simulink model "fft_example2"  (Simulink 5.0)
settings: Solver=ode45  StartTime=0.0  StopTime=10000.0  RelTol=1e-3
undefined symbols (not defined in the file or in its folder): get, hamming, N, tmp5
libraries: xbsIndex_r3 x50, xrbsControl_r3 x4, ADlibrary x3, dspsigattribs x2, dspsnks4 x2, simulink x1

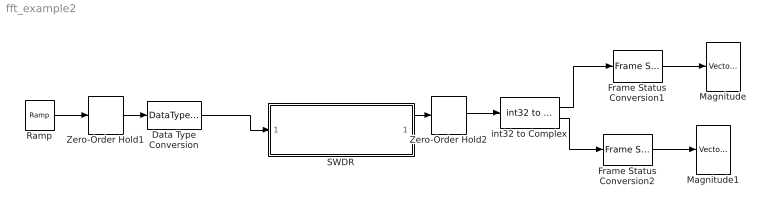
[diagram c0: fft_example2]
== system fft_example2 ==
  Data Type Conversion : DataTypeConversion  DataType=uint32
  Frame Status Conversion1 : dspsigattribs/Frame Status Conversion  growRefPort=off  outframe=Frame-based
  Frame Status Conversion2 : dspsigattribs/Frame Status Conversion  growRefPort=off  outframe=Frame-based
  Magnitude : dspsnks4/Vector Scope  ScopeProperties=on  Domain=User-defined  HorizSpan=1  DisplayProperties=off  AxisGrid=on  Memory=off  FrameNumber=on  AxisLegend=off  AxisZoom=off  OpenScopeAtSimStart=on  OpenScopeImmediately=off  FigPos=get(0,'defaultfigureposition')  AxisProperties=off  XUnits=Hertz  XRange=[0...Fs/2]  InheritXIncr=on  XIncr=1  XLabel=Frequency  YUnits=dB  YLabel=Magnitude  LineProperties=off
  Magnitude1 : dspsnks4/Vector Scope  ScopeProperties=on  Domain=User-defined  HorizSpan=1  DisplayProperties=off  AxisGrid=on  Memory=off  FrameNumber=on  AxisLegend=off  AxisZoom=off  OpenScopeAtSimStart=on  OpenScopeImmediately=off  FigPos=get(0,'defaultfigureposition')  AxisProperties=off  XUnits=Hertz  XRange=[0...Fs/2]  InheritXIncr=on  XIncr=1  XLabel=Frequency  YUnits=dB  YLabel=Magnitude  LineProperties=off
  Ramp : simulink/Sources/Ramp  slope=.02  start=0  X0=8
  SWDR : Subsystem
  Zero-Order Hold1 : ZeroOrderHold
  Zero-Order Hold2 : ZeroOrderHold  SampleTime=370
  int32 to Complex : ADlibrary/Miscellaneous/int32 to Complex
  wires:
  Frame Status Conversion1/1 -> Magnitude/1
  Ramp/1 -> Zero-Order Hold1/1
  Zero-Order Hold1/1 -> Data Type Conversion/1
  Data Type Conversion/1 -> SWDR/1(Vector Input)
  SWDR/1(Vector Output) -> Zero-Order Hold2/1
  Zero-Order Hold2/1 -> int32 to Complex/1
  Frame Status Conversion2/1 -> Magnitude1/1
  int32 to Complex/1 -> Frame Status Conversion1/1
  int32 to Complex/2 -> Frame Status Conversion2/1

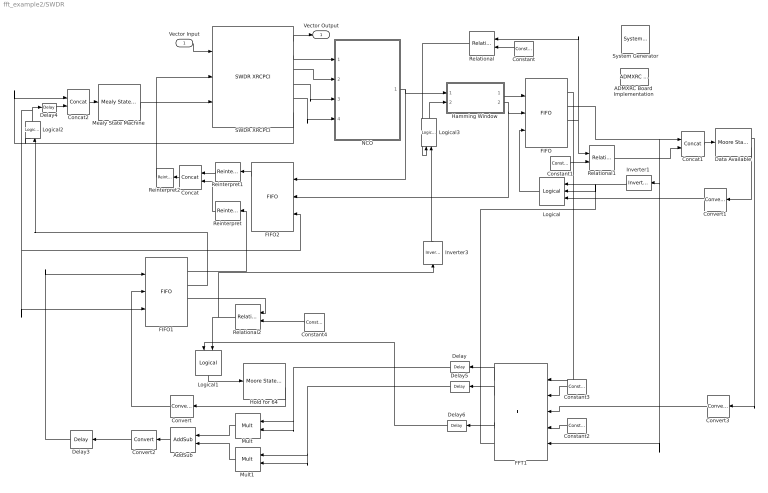
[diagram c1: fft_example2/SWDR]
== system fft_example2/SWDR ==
  Vector Input : Inport
  " System Generator" : xbsIndex_r3/ System Generator  Tag=genX  xilinxfamily=Virtex2  part=xc2v6000  speed=-4  package=ff1152  synthesis_tool=XST  directory=e:/tmp5  testbench=off  simulink_period=1  sysclk_period=15  incr_netlist=off  trim_vbits=According to Block Masks  dbl_ovrd=According to Block Masks  core_generation=According to Block Masks  run_coregen=off  deprecated_control=off  eval_field=0
  ADMXRC Board  Implementation : ADlibrary/Miscellaneous/ADMXRC Board  Implementation  board=XRCII  run_synth=on  make_clean=off  lvds_io_std=3.3v  clock_source=MCLK
  AddSub : xbsIndex_r3/AddSub  Orientation=left  mode=Addition  precision=Full  arith_type=Unsigned  n_bits=8  bin_pt=2  quantization=Truncate  overflow=Wrap  latency=0  explicit_period=off  period=1  en=off  dbl_ovrd=off  use_core=on  pipeline=off  use_rpm=off  gen_core=on
  Concat : xbsIndex_r3/Concat  Orientation=left  num_inputs=2  explicit_period=off  period=1  dbl_ovrd=off
  Concat1 : xbsIndex_r3/Concat  num_inputs=2  explicit_period=off  period=1  dbl_ovrd=off
  Concat2 : xbsIndex_r3/Concat  num_inputs=2  explicit_period=off  period=1  dbl_ovrd=off
  Constant : xbsIndex_r3/Constant  Orientation=left  const=.75  arith_type=Unsigned  n_bits=3  bin_pt=3  explicit_period=off  period=1  dbl_ovrd=off
  Constant1 : xbsIndex_r3/Constant  const=.25  arith_type=Unsigned  n_bits=3  bin_pt=3  explicit_period=off  period=1  dbl_ovrd=off
  Constant2 : xbsIndex_r3/Constant  Orientation=left  const=0  arith_type=Boolean  n_bits=1  bin_pt=0  explicit_period=on  period=1  dbl_ovrd=off
  Constant3 : xbsIndex_r3/Constant  Orientation=left  const=0  arith_type="Signed  (2's comp)"  n_bits=16  bin_pt=0  explicit_period=on  period=1  dbl_ovrd=off
  Constant4 : xbsIndex_r3/Constant  Orientation=left  const=.7  arith_type=Unsigned  n_bits=5  bin_pt=5  explicit_period=off  period=1  dbl_ovrd=off
  Convert : xbsIndex_r3/Convert  Orientation=left  arith_type=Boolean  n_bits=8  bin_pt=6  quantization=Truncate  overflow=Wrap  latency=0  explicit_period=off  period=1  dbl_ovrd=off  inserted_by_tool=off
  Convert1 : xbsIndex_r3/Convert  Orientation=left  arith_type=Boolean  n_bits=8  bin_pt=6  quantization=Truncate  overflow=Wrap  latency=0  explicit_period=off  period=1  dbl_ovrd=off  inserted_by_tool=off
  Convert2 : xbsIndex_r3/Convert  Orientation=left  arith_type="Signed  (2's comp)"  n_bits=16  bin_pt=0  quantization=Truncate  overflow=Wrap  latency=0  explicit_period=off  period=1  dbl_ovrd=off  inserted_by_tool=off
  Convert3 : xbsIndex_r3/Convert  Orientation=left  arith_type=Boolean  n_bits=8  bin_pt=6  quantization=Truncate  overflow=Wrap  latency=0  explicit_period=off  period=1  dbl_ovrd=off  inserted_by_tool=off
  Data Available : xrbsControl_r3/Moore State Machine  next_state_matrix=[0 1 0 1;1 1 0 0]  output_matrix=[0;1]  n_bits=1  period=1
  Delay : xbsIndex_r3/Delay  Orientation=left  latency=1  reg_retiming=off  explicit_period=on  period=1  en=off  accept_only_valid=off  init_zero=on  dbl_ovrd=off
  Delay3 : xbsIndex_r3/Delay  Orientation=left  latency=1  reg_retiming=off  explicit_period=on  period=1  en=off  accept_only_valid=off  init_zero=on  dbl_ovrd=off
  Delay4 : xbsIndex_r3/Delay  latency=1  reg_retiming=off  explicit_period=on  period=1  en=off  accept_only_valid=off  init_zero=on  dbl_ovrd=off
  Delay5 : xbsIndex_r3/Delay  Orientation=left  latency=1  reg_retiming=off  explicit_period=on  period=1  en=off  accept_only_valid=off  init_zero=on  dbl_ovrd=off
  Delay6 : xbsIndex_r3/Delay  Orientation=left  latency=2  reg_retiming=off  explicit_period=on  period=1  en=off  accept_only_valid=off  init_zero=on  dbl_ovrd=off
  FFT1 : xbsIndex_r3/FFT  Orientation=left  n=64  mem=Single  scale_mode=1/N  oflw_inv=off  explicit_period=on  period=1  rst=on  dbl_ovrd=off  gen_core=on
  FIFO : xbsIndex_r3/FIFO  depth=256  percent_nbits=3  mem_type=Block RAM  store_only_valid=on  init_zero=on  explicit_period=on  period=1  rst=off  en=off  dbl_ovrd=off  gen_core=on
  FIFO1 : xbsIndex_r3/FIFO  depth=512  percent_nbits=5  mem_type=Block RAM  store_only_valid=off  init_zero=on  explicit_period=on  period=1  rst=off  en=off  dbl_ovrd=off  gen_core=on
  FIFO2 : xbsIndex_r3/FIFO  Orientation=left  depth=1K  percent_nbits=3  mem_type=Block RAM  store_only_valid=on  init_zero=on  explicit_period=on  period=1  rst=off  en=off  dbl_ovrd=off  gen_core=on
  Hamming Window : Subsystem
  Hold for 64 : xrbsControl_r3/Moore State Machine  next_state_matrix=[0 1;[(2:64)' (2:64)']; 0 0]  output_matrix=[0;ones(64,1)]  n_bits=1  period=1
  Inverter1 : xbsIndex_r3/Inverter  Orientation=left  latency=0  explicit_period=off  period=1  en=off  dbl_ovrd=off
  Inverter3 : xbsIndex_r3/Inverter  Orientation=up  latency=0  explicit_period=off  period=1  en=off  dbl_ovrd=off
  Logical : xbsIndex_r3/Logical  Orientation=left  logical_function=AND  inputs=3  precision=Full  arith_type=Unsigned  n_bits=8  bin_pt=2  align_bp=on  latency=0  explicit_period=off  period=1  en=off  dbl_ovrd=off
  Logical1 : xbsIndex_r3/Logical  Orientation=down  logical_function=AND  inputs=2  precision=Full  arith_type=Unsigned  n_bits=8  bin_pt=2  align_bp=on  latency=0  explicit_period=off  period=1  en=off  dbl_ovrd=off
  Logical2 : xbsIndex_r3/Logical  Orientation=up  logical_function=NOR  inputs=2  precision=Full  arith_type=Unsigned  n_bits=8  bin_pt=2  align_bp=on  latency=0  explicit_period=off  period=1  en=off  dbl_ovrd=off
  Logical3 : xbsIndex_r3/Logical  Orientation=up  logical_function=OR  inputs=2  precision=Full  arith_type=Unsigned  n_bits=8  bin_pt=2  align_bp=on  latency=0  explicit_period=off  period=1  en=off  dbl_ovrd=off
  Mealy State Machine : xrbsControl_r3/Mealy State Machine  next_state_matrix=[0 0 1 1; 0 0 1 1]  output_matrix=[0 1 0 0; 1 1 0 0]  n_bits=1  period=1
  Mult : xbsIndex_r3/Mult  Orientation=left  precision=Full  arith_type="Signed  (2's comp)"  n_bits=16  bin_pt=0  quantization=Truncate  overflow=Wrap  mult_type=Parallel  use_embedded=off  pipeline=off  latency=1  explicit_period=off  period=1  en=off  dbl_ovrd=off  oversample=2  use_rpm=off  placement_style=Rectangular Shape  gen_core=on
  Mult1 : xbsIndex_r3/Mult  Orientation=left  precision=Full  arith_type="Signed  (2's comp)"  n_bits=16  bin_pt=0  quantization=Truncate  overflow=Wrap  mult_type=Parallel  use_embedded=off  pipeline=off  latency=1  explicit_period=off  period=1  en=off  dbl_ovrd=off  oversample=2  use_rpm=off  placement_style=Rectangular Shape  gen_core=on
  NCO : Subsystem
  Reinterpret : xbsIndex_r3/Reinterpret  Orientation=left  force_arith_type=on  arith_type=Unsigned  force_bin_pt=on  bin_pt=0  force_valid=off
  Reinterpret1 : xbsIndex_r3/Reinterpret  Orientation=left  force_arith_type=on  arith_type=Unsigned  force_bin_pt=on  bin_pt=0  force_valid=off
  Reinterpret2 : xbsIndex_r3/Reinterpret  Orientation=left  force_arith_type=on  arith_type="Signed  (2's comp)"  force_bin_pt=on  bin_pt=0  force_valid=off
  Relational : xbsIndex_r3/Relational  Orientation=left  mode=a>=b  latency=0  explicit_period=off  period=1  en=off  dbl_ovrd=off
  Relational1 : xbsIndex_r3/Relational  mode=a>=b  latency=0  explicit_period=off  period=1  en=off  dbl_ovrd=off
  Relational2 : xbsIndex_r3/Relational  Orientation=left  mode=a<b  latency=0  explicit_period=off  period=1  en=off  dbl_ovrd=off
  SWDR XRCPCI : ADlibrary/PCI/SWDR XRCPCI  AncestorBlock=ADlibrary/PCI/ADMA XRCPCI  no_inputs=1  no_outputs=64  circuit_lag=192  fifo_length=256  debug=0
  Vector Output : Outport
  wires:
  SWDR XRCPCI/1 -> Vector Output/1
  Vector Input/1 -> SWDR XRCPCI/1
  SWDR XRCPCI/2 -> NCO/1(data)
  SWDR XRCPCI/3 -> NCO/2(addr)
  SWDR XRCPCI/5 -> NCO/4(reset)
  NCO/1(sine) -> Hamming Window/1(data), FIFO2/1
  Hamming Window/1(wdata) -> FIFO/1
  Constant/1 -> Relational/2
  Constant1/1 -> Relational1/2
  FIFO/2 -> Concat1/1, Inverter1/1, FFT1/5
  Inverter1/1 -> Logical/1
  Mult/1 -> AddSub/1
  Mult1/1 -> AddSub/2
  AddSub/1 -> Convert2/1
  Delay3/1 -> FIFO1/1
  Logical1/1 -> Hold for 64/1
  Constant4/1 -> Relational2/2
  Delay6/1 -> Logical1/1
  FIFO1/1 -> Reinterpret/1
  Reinterpret1/1 -> Concat/1
  Reinterpret/1 -> Concat/2
  Concat/1 -> Reinterpret2/1
  Relational1/1 -> Concat1/2
  Concat1/1 -> Data Available/1
  Data Available/2 -> Convert1/1
  Logical3/1 -> Hamming Window/2(wait)
  Inverter3/1 -> Logical3/2
  Relational/1 -> Logical3/1
  SWDR XRCPCI/4 -> NCO/3(write)
  Hamming Window/2(write) -> FIFO/2, FIFO2/2
  Logical/1 -> FIFO/3
  Reinterpret2/1 -> SWDR XRCPCI/2
  FIFO2/1 -> Reinterpret1/1
  Concat2/1 -> Mealy State Machine/1
  Mealy State Machine/2 -> SWDR XRCPCI/3
  SWDR XRCPCI/6 -> Concat2/1, Logical2/1
  Delay4/1 -> Concat2/2
  Logical2/1 -> Delay4/1, FIFO1/3, FIFO2/3
  Convert2/1 -> Delay3/1
  FIFO1/3 -> Relational2/1
  Relational2/1 -> Logical1/2, Inverter3/1
  Hold for 64/2 -> Convert/1
  FIFO/3 -> Relational/1, Relational1/1
  FFT1/1 -> Delay/1
  FFT1/2 -> Delay5/1
  FFT1/4 -> Delay6/1
  FFT1/5 -> Logical/2
  Constant3/1 -> FFT1/2
  FIFO/1 -> FFT1/1
  Constant2/1 -> FFT1/4
  Data Available/1 -> Convert3/1
  FIFO1/2 -> Logical2/2
  Delay/1 -> Mult/1, Mult/2
  Delay5/1 -> Mult1/1, Mult1/2
  Convert/1 -> FIFO1/2
  Convert1/1 -> Logical/3
  Convert3/1 -> FFT1/3

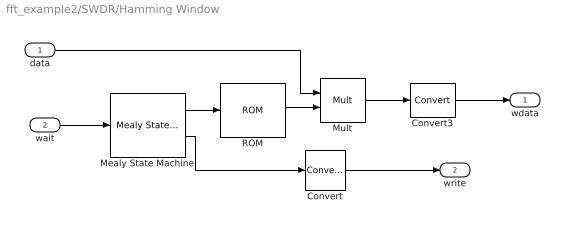
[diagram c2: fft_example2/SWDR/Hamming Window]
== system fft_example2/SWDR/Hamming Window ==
  data : Inport
  wait : Inport  Port=2
  Convert : xbsIndex_r3/Convert  arith_type=Boolean  n_bits=8  bin_pt=6  quantization=Truncate  overflow=Wrap  latency=0  explicit_period=off  period=1  dbl_ovrd=off  inserted_by_tool=off
  Convert3 : xbsIndex_r3/Convert  arith_type="Signed  (2's comp)"  n_bits=16  bin_pt=0  quantization=Truncate  overflow=Wrap  latency=0  explicit_period=on  period=1  dbl_ovrd=off  inserted_by_tool=off
  Mealy State Machine : xrbsControl_r3/Mealy State Machine  next_state_matrix=[1 0;[(2:63)' (2:63)'];0 0]  output_matrix=[1 0;ones(63,2)]  n_bits=1  period=1
  Mult : xbsIndex_r3/Mult  precision=Full  arith_type="Signed  (2's comp)"  n_bits=8  bin_pt=2  quantization=Truncate  overflow=Wrap  mult_type=Parallel  use_embedded=off  pipeline=off  latency=0  explicit_period=on  period=1  en=off  dbl_ovrd=off  oversample=2  use_rpm=off  placement_style=Rectangular Shape  gen_core=on
  ROM : xbsIndex_r3/ROM  depth=64  initVector=hamming(64)  arith_type="Signed  (2's comp)"  n_bits=16  bin_pt=16  latency=1  distributed_mem=off  init_zero=on  explicit_period=on  period=1  rst=off  init_reg=0  en=off  dbl_ovrd=off  use_rpm=off  gen_core=on
  wdata : Outport
  write : Outport  Port=2
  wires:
  wait/1 -> Mealy State Machine/1
  Mealy State Machine/1 -> ROM/1
  ROM/1 -> Mult/2
  data/1 -> Mult/1
  Mult/1 -> Convert3/1
  Mealy State Machine/2 -> Convert/1
  Convert3/1 -> wdata/1
  Convert/1 -> write/1

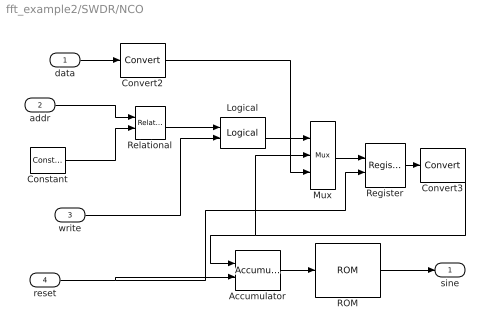
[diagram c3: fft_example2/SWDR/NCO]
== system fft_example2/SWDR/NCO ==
  data : Inport
  addr : Inport  Port=2
  write : Inport  Port=3
  reset : Inport  Port=4
  Accumulator : xbsIndex_r3/Accumulator  n_bits=10  overflow=Wrap  operation=Add  scale=1  explicit_period=off  period=1  rst=on  hasbypass=on  en=off  dbl_ovrd=off  gen_core=on  use_rpm=off
  Constant : xbsIndex_r3/Constant  const=0  arith_type=Unsigned  n_bits=22  bin_pt=0  explicit_period=on  period=1  dbl_ovrd=off
  Convert2 : xbsIndex_r3/Convert  arith_type=Unsigned  n_bits=10  bin_pt=0  quantization=Truncate  overflow=Wrap  latency=0  explicit_period=on  period=1  dbl_ovrd=off  inserted_by_tool=off
  Convert3 : xbsIndex_r3/Convert  arith_type=Unsigned  n_bits=10  bin_pt=0  quantization=Truncate  overflow=Wrap  latency=0  explicit_period=on  period=1  dbl_ovrd=off  inserted_by_tool=off
  Logical : xbsIndex_r3/Logical  logical_function=AND  inputs=2  precision=Full  arith_type=Unsigned  n_bits=8  bin_pt=2  align_bp=on  latency=0  explicit_period=on  period=1  en=off  dbl_ovrd=off
  Mux : xbsIndex_r3/Mux  inputs=2  precision=Full  arith_type="Signed  (2's comp)"  n_bits=8  bin_pt=2  quantization=Truncate  overflow=Wrap  latency=0  mux_type=off  explicit_period=on  period=1  en=off  dbl_ovrd=off  use_rpm=off  gen_core=on
  ROM : xbsIndex_r3/ROM  depth=1024  initVector=256*sin(2*pi*(0:1023)/1024)  arith_type="Signed  (2's comp)"  n_bits=16  bin_pt=0  latency=1  distributed_mem=off  init_zero=on  explicit_period=on  period=1  rst=off  init_reg=0  en=off  dbl_ovrd=off  use_rpm=off  gen_core=on
  Register : xbsIndex_r3/Register  init=0  reg_only_valid=on  explicit_period=on  period=1  rst=on  en=off  out_en=off  dbl_ovrd=off
  Relational : xbsIndex_r3/Relational  mode=a=b  latency=0  explicit_period=on  period=1  en=off  dbl_ovrd=off
  sine : Outport
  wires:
  Accumulator/1 -> ROM/1
  data/1 -> Convert2/1
  Register/1 -> Convert3/1
  Mux/1 -> Register/1
  Convert3/1 -> Accumulator/1, Mux/2
  Convert2/1 -> Mux/3
  Logical/1 -> Mux/1
  write/1 -> Logical/2
  Constant/1 -> Relational/2
  addr/1 -> Relational/1
  ROM/1 -> sine/1
  reset/1 -> Accumulator/2, Register/2
  Relational/1 -> Logical/1
